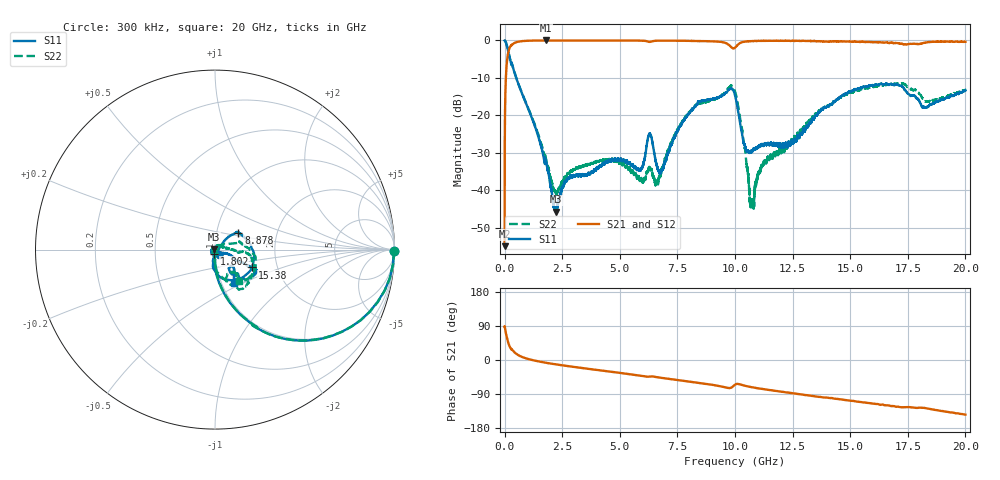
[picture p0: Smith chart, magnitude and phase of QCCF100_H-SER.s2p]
! Created Mon Feb  8 13:52:58 2021
# hz S ma R 50
! 2 Port Network Data from SP1.SP block
! freq  magS11  angS11  magS21  angS21  magS12  angS12  magS22  angS22
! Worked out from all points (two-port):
!   20001 points, 300 kHz to 20 GHz, reference 50 ohm
!   highest |S21| = -0.01 dB at 1.809 GHz (marker M1); lowest = -55.0 dB at 300 kHz (marker M2)
!   |S21| within 3 dB of the highest: 164.7 MHz to end of sweep
!   lowest |S11| = -45.7 dB at 2.223 GHz (marker M3), VSWR 1.01, Z = 49.5 + j0.113 ohm
!   |S11| at or under -10 dB: 505.5 MHz to end of sweep
!   |S22| runs from -45.0 to 0.0 dB; largest |S21 - S12| = 0.013
!   S11 on the Smith chart (normalised r, x): 300 kHz: open; 1.802 GHz: 0.99, -0.04; 8.878 GHz: 1.27, +0.25; 15.38 GHz: 1.48, -0.31; 20 GHz: 1.15, -0.45
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300000  0.997 -0.4  0.001787 88.5  0.001787 90.7  0.9988 -0.4
1.043e8  0.8417 -33.0  0.5349 57.3  0.5357 57.3  0.843 -32.9
2.113e8  0.6085 -53.7  0.7889 36.8  0.7879 36.8  0.6075 -53.8
6.263e8  0.249 -78.2  0.9669 11.8  0.9678 11.8  0.25 -77.9
1.8023e9  0.02356 -105.3  0.9982 -7.4  0.9984 -7.4  0.02575 -85.4
1.8093e9  0.02297 -105.9  0.9987 -7.5  0.9977 -7.5  0.02526 -85.0
2.2233e9  0.005179 167.3  0.9978 -11.5  0.9974 -11.5  0.009428 -28.1
3.3343e9  0.01545 140.0  0.9963 -20.9  0.9969 -20.9  0.02075 -13.2
5.8923e9  0.01858 -61.1  0.9949 -41.3  0.9952 -41.2  0.0137 149.4
6.2983e9  0.057 -49.6  0.9571 -43.6  0.9573 -43.6  0.01963 -44.7
6.6673e9  0.01844 -45.7  0.9924 -45.8  0.9927 -45.8  0.01274 118.1
7.6633e9  0.07455 43.1  0.9909 -54.1  0.9904 -54.1  0.07764 23.8
8.8783e9  0.1613 36.0  0.9751 -64.2  0.9757 -64.3  0.1547 10.8
1.00003e10  0.1845 -66.2  0.8001 -65.1  0.7997 -65.1  0.208 -60.6
1.04243e10  0.03978 -92.8  0.9646 -67.9  0.9643 -67.9  0.03666 -92.7
1.07353e10  0.03353 -60.5  0.9802 -72.0  0.9807 -71.9  0.007044 2.0
1.12293e10  0.04001 -55.9  0.9871 -77.0  0.9886 -77.0  0.02242 60.6
1.33343e10  0.08479 -18.9  0.982 -94.6  0.9825 -94.7  0.09201 0.0
1.53783e10  0.2294 -25.7  0.9572 -110.3  0.9574 -110.2  0.2137 -16.2
1.66673e10  0.2553 -29.6  0.9247 -119.9  0.9301 -120.4  0.2573 -41.3
1.82123e10  0.1285 -49.5  0.929 -126.4  0.9267 -126.4  0.1572 -64.1
2e10  0.2148 -60.1  0.9596 -144.2  0.9538 -144.1  0.2192 -52.8
